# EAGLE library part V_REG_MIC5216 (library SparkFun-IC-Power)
500mA LDO, MSOP8 for better dissipation
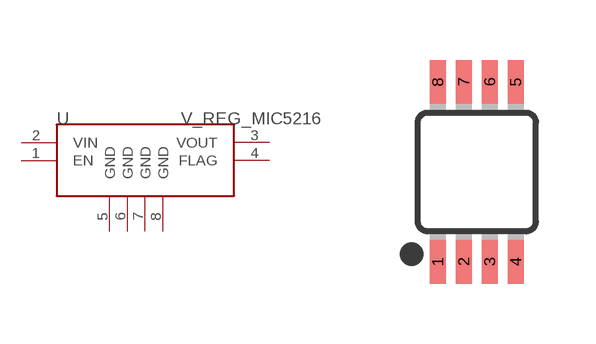
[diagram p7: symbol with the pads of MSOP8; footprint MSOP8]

Designator prefix U

## V_REG_MIC5216 (PROD_ID: IC-09527)  [MSOP8]
1  EN
2  VIN
3  VOUT
4  FLAG
5  GND
6  GND
7  GND
8  GND

## Footprint MSOP8 (pad centres in mm)
8M, 8-Lead, 0.118" Wide, Miniature Small Outline Package MSOP 8M-Package doc1097.pdf
smd 0.4 x 1.1: 1 -0.975,-2.25; 2 -0.325,-2.25; 3 0.325,-2.25; 4 0.975,-2.25; 5 0.975,2.25; 6 0.325,2.25; 7 -0.325,2.25; 8 -0.975,2.25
